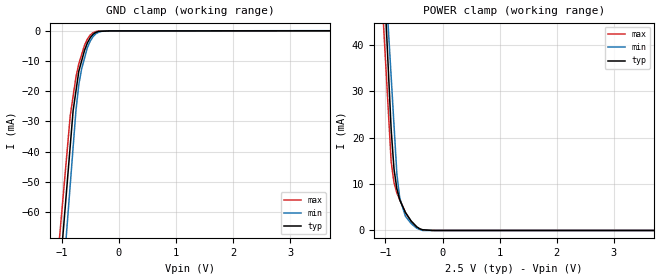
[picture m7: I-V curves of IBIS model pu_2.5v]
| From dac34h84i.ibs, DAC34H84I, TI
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[Model] pu_2.5v
Model_type Input
Vinl = 750.000mV
Vinh = 1.75000V
C_comp 609.000fF 588.000fF 630.000fF
| variable typ   min   max
[Voltage Range] 2.50000V 2.25000V 2.75000V
[POWER Clamp Reference] 2.50000V 2.25000V 2.75000V
[GND Clamp Reference] 0.00000V 0.00000V 0.00000V
[Temperature Range] 25   125   -40
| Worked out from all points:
|   GND clamp passes 1 mA (typ) near -0.44 V on its own axis
|   POWER clamp passes 1 mA (typ) near -0.47 V on its own axis
[GND Clamp]
-2.5V     -419.3mA   -455.9mA   -383.2mA
-850mV    -37.99mA   -50.86mA   -28.04mA
-800mV    -26.43mA   -38.58mA   -21.65mA
-750mV    -19.9mA    -26.31mA   -15.25mA
-700mV    -13.36mA   -17.75mA   -10.86mA
-650mV    -9.906mA   -12.54mA   -7.818mA
-600mV    -6.455mA   -9.035mA   -4.776mA
-550mV    -3.994mA   -5.529mA   -2.711mA
-450mV    -1.129mA   -1.893mA   -591.7uA
-350mV    -176.7uA   -404.1uA   -69.67uA
-150mV    -19.8uA    -18.84uA   -24.67uA
5V        43.63uA    97.51uA    26.2uA
[POWER Clamp]
-2.5V     437.9mA    368.4mA    368mA
-1.05V    60.82mA    64.59mA    47.96mA
-900mV    21.81mA    33.16mA    14.86mA
-850mV    13.24mA    22.68mA    10.31mA
-800mV    9.004mA    12.2mA     8.082mA
-750mV    6.595mA    7.025mA    6.669mA
-650mV    3.89mA     3.07mA     3.845mA
-550mV    2.037mA    1.496mA    1.954mA
-450mV    776uA      475.6uA    629.5uA
-350mV    158.4uA    0A         74.18uA
-175mV    0A         0A         30.91uA
5V        0A         0A         0A
